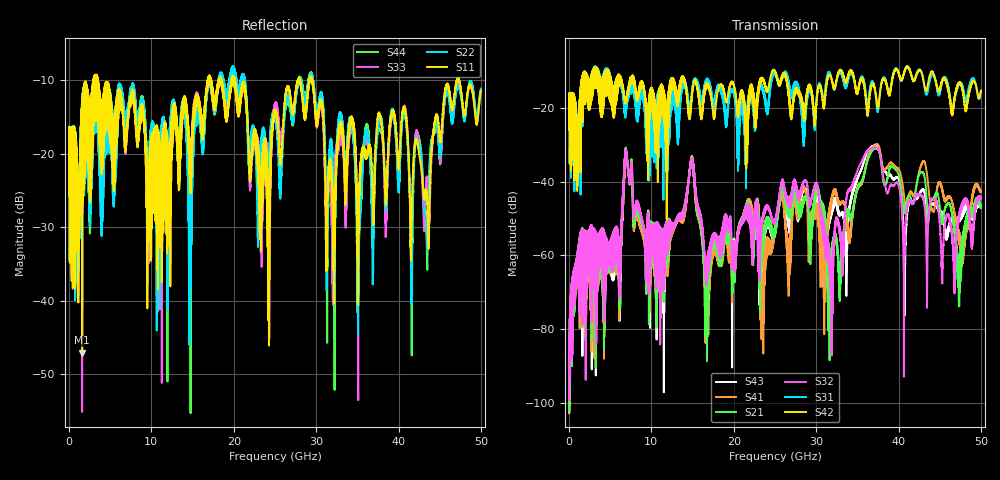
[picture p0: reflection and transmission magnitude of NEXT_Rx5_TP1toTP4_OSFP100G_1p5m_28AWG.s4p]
! Touchstone data
! Created: 27-Feb-2019 by IdEM 12 (12.1.0)
! COMMENTS
!  Created Wed Feb 27 09:43:39 2019
!  64 Port Network Data from SP1.SP block
!  freq  magS1_1  angS1_1  magS1_2  angS1_2  magS1_3  angS1_3  magS1_4  angS1_4
!  magS1_5  angS1_5  magS1_6  angS1_6  magS1_7  angS1_7  magS1_8  angS1_8
!  magS1_9  angS1_9  magS1_10  angS1_10  magS1_11  angS1_11  magS1_12  angS1_12
!  magS1_13  angS1_13  magS1_14  angS1_14  magS1_15  angS1_15  magS1_16  angS1_16
!  magS1_17  angS1_17  magS1_18  angS1_18  magS1_19  angS1_19  magS1_20  angS1_20
!  magS1_21  angS1_21  magS1_22  angS1_22  magS1_23  angS1_23  magS1_24  angS1_24
!  magS1_25  angS1_25  magS1_26  angS1_26  magS1_27  angS1_27  magS1_28  angS1_28
!  magS1_29  angS1_29  magS1_30  angS1_30  magS1_31  angS1_31  magS1_32  angS1_32
!  magS1_33  angS1_33  magS1_34  angS1_34  magS1_35  angS1_35  magS1_36  angS1_36
!  magS1_37  angS1_37  magS1_38  angS1_38  magS1_39  angS1_39  magS1_40  angS1_40
!  magS1_41  angS1_41  magS1_42  angS1_42  magS1_43  angS1_43  magS1_44  angS1_44
!  magS1_45  angS1_45  magS1_46  angS1_46  magS1_47  angS1_47  magS1_48  angS1_48
!  magS1_49  angS1_49  magS1_50  angS1_50  magS1_51  angS1_51  magS1_52  angS1_52
!  magS1_53  angS1_53  magS1_54  angS1_54  magS1_55  angS1_55  magS1_56  angS1_56
!  magS1_57  angS1_57  magS1_58  angS1_58  magS1_59  angS1_59  magS1_60  angS1_60
!  magS1_61  angS1_61  magS1_62  angS1_62  magS1_63  angS1_63  magS1_64  angS1_64
!  magS2_1  angS2_1  magS2_2  angS2_2  magS2_3  angS2_3  magS2_4  angS2_4
!  magS2_5  angS2_5  magS2_6  angS2_6  magS2_7  angS2_7  magS2_8  angS2_8
!  magS2_9  angS2_9  magS2_10  angS2_10  magS2_11  angS2_11  magS2_12  angS2_12
!  magS2_13  angS2_13  magS2_14  angS2_14  magS2_15  angS2_15  magS2_16  angS2_16
!  magS2_17  angS2_17  magS2_18  angS2_18  magS2_19  angS2_19  magS2_20  angS2_20
!  magS2_21  angS2_21  magS2_22  angS2_22  magS2_23  angS2_23  magS2_24  angS2_24
!  magS2_25  angS2_25  magS2_26  angS2_26  magS2_27  angS2_27  magS2_28  angS2_28
!  magS2_29  angS2_29  magS2_30  angS2_30  magS2_31  angS2_31  magS2_32  angS2_32
!  magS2_33  angS2_33  magS2_34  angS2_34  magS2_35  angS2_35  magS2_36  angS2_36
!  magS2_37  angS2_37  magS2_38  angS2_38  magS2_39  angS2_39  magS2_40  angS2_40
!  magS2_41  angS2_41  magS2_42  angS2_42  magS2_43  angS2_43  magS2_44  angS2_44
!  magS2_45  angS2_45  magS2_46  angS2_46  magS2_47  angS2_47  magS2_48  angS2_48
!  magS2_49  angS2_49  magS2_50  angS2_50  magS2_51  angS2_51  magS2_52  angS2_52
!  magS2_53  angS2_53  magS2_54  angS2_54  magS2_55  angS2_55  magS2_56  angS2_56
!  magS2_57  angS2_57  magS2_58  angS2_58  magS2_59  angS2_59  magS2_60  angS2_60
!  magS2_61  angS2_61  magS2_62  angS2_62  magS2_63  angS2_63  magS2_64  angS2_64
!  magS3_1  angS3_1  magS3_2  angS3_2  magS3_3  angS3_3  magS3_4  angS3_4
!  magS3_5  angS3_5  magS3_6  angS3_6  magS3_7  angS3_7  magS3_8  angS3_8
!  magS3_9  angS3_9  magS3_10  angS3_10  magS3_11  angS3_11  magS3_12  angS3_12
!  magS3_13  angS3_13  magS3_14  angS3_14  magS3_15  angS3_15  magS3_16  angS3_16
!  magS3_17  angS3_17  magS3_18  angS3_18  magS3_19  angS3_19  magS3_20  angS3_20
!  magS3_21  angS3_21  magS3_22  angS3_22  magS3_23  angS3_23  magS3_24  angS3_24
!  magS3_25  angS3_25  magS3_26  angS3_26  magS3_27  angS3_27  magS3_28  angS3_28
!  magS3_29  angS3_29  magS3_30  angS3_30  magS3_31  angS3_31  magS3_32  angS3_32
!  magS3_33  angS3_33  magS3_34  angS3_34  magS3_35  angS3_35  magS3_36  angS3_36
!  magS3_37  angS3_37  magS3_38  angS3_38  magS3_39  angS3_39  magS3_40  angS3_40
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# Hz S MA R 50
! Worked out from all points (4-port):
!   5000 points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, 10 MHz to 50 GHz, reference 50 ohm
!   strongest paths, dB at 10 MHz, 12.51 GHz, 25.01 GHz, 37.51 GHz, 50 GHz:
!     S42: -19.6, -13.2, -10.0, -20.0, -15.2
!     S31: -19.6, -16.2, -10.8, -21.0, -15.4
!     S32: -94.8, -51.4, -50.6, -31.1, -44.8
!     S21: -96.5, -51.2, -52.7, -31.3, -46.4
!     S41: -97.0, -51.8, -52.7, -29.9, -42.9
!     S43: -96.7, -51.8, -53.0, -30.4, -46.3
!   lowest |S11| = -47.1 dB at 1.59 GHz (marker M1), VSWR 1.01, Z = 49.7 + j0.298 ohm
!   |S11| at or under -10 dB: 3.482 GHz to 16.85 GHz (13.37 GHz wide, 132 % of centre); 20.15 GHz to 27.79 GHz (7.635 GHz wide, 31.9 % of centre); 29.53 GHz to 47.08 GHz (17.55 GHz wide, 45.8 % of centre)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
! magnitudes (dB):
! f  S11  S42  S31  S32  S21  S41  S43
! 10 MHz  -19.2  -19.6  -19.6  -94.8  -96.5  -97.0  -96.7
! 1.59 GHz  -47.1  -23.5  -24.2  -56.7  -56.5  -57.8  -57.2
! 6.95 GHz  -18.5  -18.1  -20.2  -31.6  -31.2  -31.9  -32.3
! 14.94 GHz  -17.3  -16.0  -15.1  -33.6  -33.4  -33.4  -33.2
! 16.75 GHz  -10.8  -13.6  -12.8  -66.5  -88.7  -66.5  -75.2
! 37.09 GHz  -24.1  -14.3  -14.3  -30.7  -31.0  -30.0  -30.1
! 50 GHz  -11.5  -15.2  -15.4  -44.8  -46.4  -42.9  -46.3
